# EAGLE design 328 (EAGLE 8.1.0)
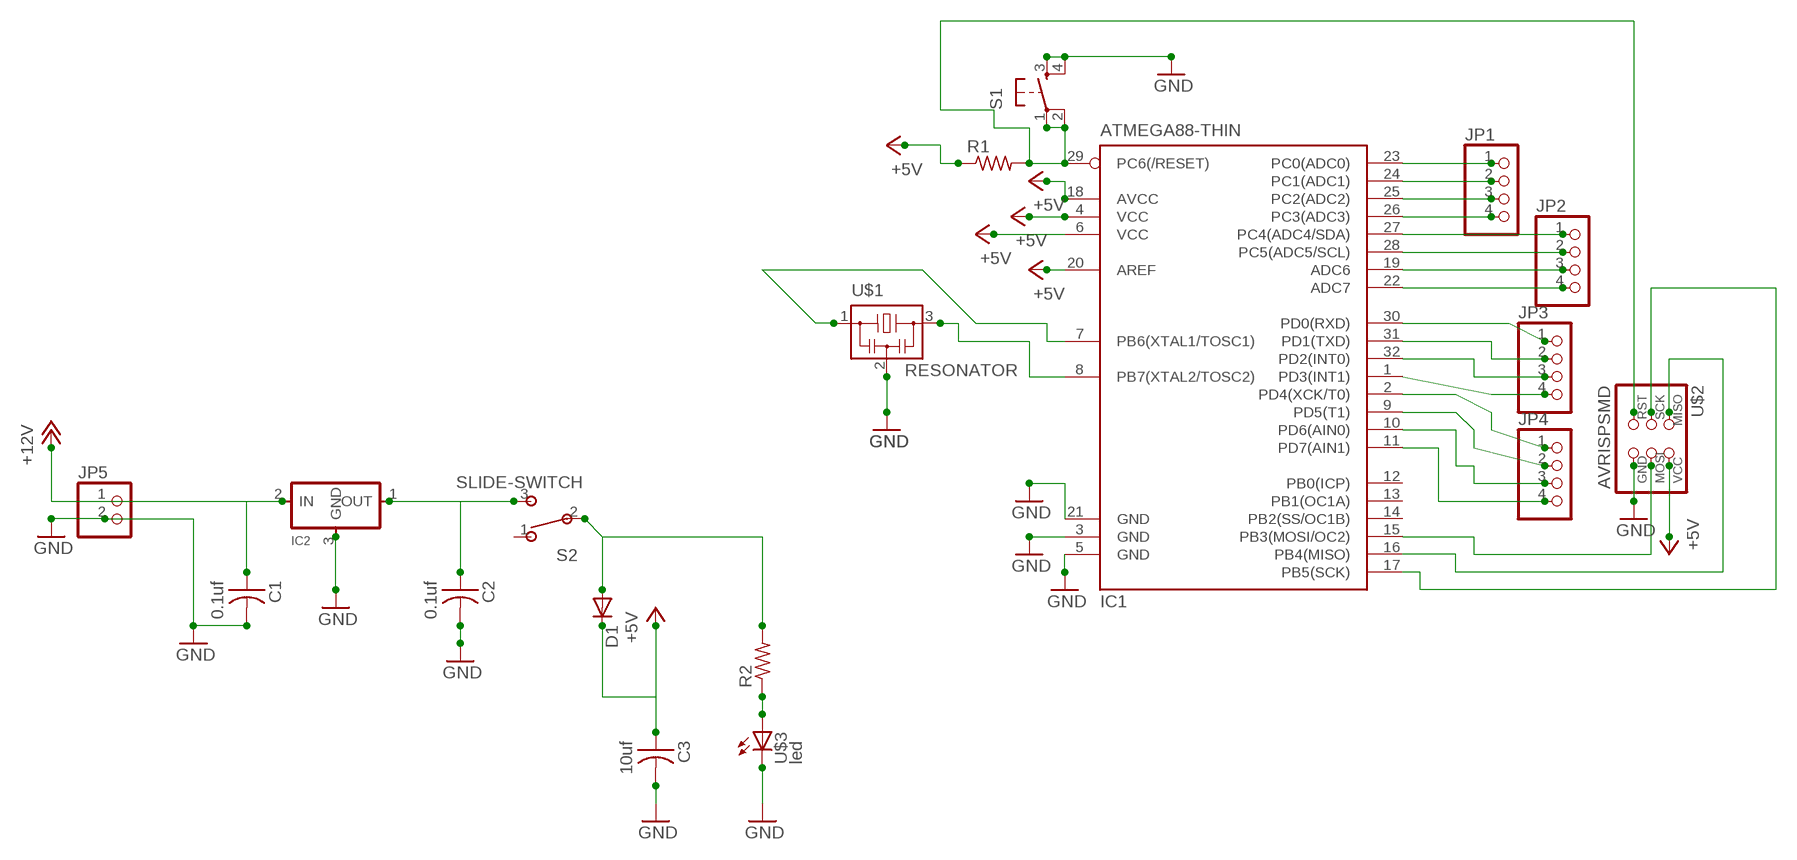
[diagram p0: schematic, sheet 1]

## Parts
C1  0.1uf  CAP-US1206FAB  [C1206FAB]
C2  0.1uf  CAP-US1206FAB  [C1206FAB]
C3  10uf  CAP-US1206FAB  [C1206FAB]
D1  DIODESOD123  [SOD123]
IC1  ATMEGA88-THIN  [TQFP32-08THIN]
IC2  REGULATORSOT23  [SOT23]
JP1  PINHD-1X4  [1X04]
JP2  PINHD-1X4  [1X04]
JP3  PINHD-1X4  [1X04]
JP4  PINHD-1X4  [1X04]
JP5  PINHD-1X2  [1X02]
R1  RES-US1206FAB  [R1206FAB]
R2  RES-US1206FAB  [R1206FAB]
S1  6MM_SWITCH6MM_SWITCH  [6MM_SWITCH]
S2  SLIDE-SWITCH  [AYZ0102AGRLC]
U$1  RESONATOR  [EFOBM]
U$2  AVRISPSMD  [2X03SMD]
U$3  led  LEDFAB1206  [LED1206FAB]

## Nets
+5V: C3.1 D1.CATHODE(C) IC1.4(VCC) IC1.6(VCC) IC1.18(AVCC) IC1.20(AREF) R1.1 U$2.2(VCC)
+12V: C1.1 IC2.2(IN) JP5.1
GND: C1.2 C2.2 C3.2 IC1.3(GND) IC1.5(GND) IC1.21(GND) IC2.3(GND) JP5.2 S1.3(S) S1.4(S1) U$1.2 U$2.6(GND) U$3.2(C)
N$1: IC1.7(PB6(XTAL1/TOSC1)) U$1.1
N$2: IC1.8(PB7(XTAL2/TOSC2)) U$1.3
N$3: IC1.29(PC6(/RESET)) R1.2 S1.1(P) S1.2(P1) U$2.5(RST)
N$4: IC1.17(PB5(SCK)) U$2.3(SCK)
N$5: IC1.16(PB4(MISO)) U$2.1(MISO)
N$6: IC1.15(PB3(MOSI/OC2)) U$2.4(MOSI)
N$7: IC1.23(PC0(ADC0)) JP1.1
N$8: IC1.24(PC1(ADC1)) JP1.2
N$9: IC1.25(PC2(ADC2)) JP1.3
N$10: IC1.26(PC3(ADC3)) JP1.4
N$11: IC1.27(PC4(ADC4/SDA)) JP2.1
N$12: IC1.28(PC5(ADC5/SCL)) JP2.2
N$13: IC1.19(ADC6) JP2.3
N$14: IC1.22(ADC7) JP2.4
N$15: IC1.30(PD0(RXD)) JP3.1
N$16: IC1.31(PD1(TXD)) JP3.2
N$17: IC1.32(PD2(INT0)) JP3.3
N$18: IC1.1(PD3(INT1)) JP3.4
N$19: IC1.2(PD4(XCK/T0)) JP4.1
N$20: IC1.9(PD5(T1)) JP4.2
N$21: IC1.10(PD6(AIN0)) JP4.3
N$22: IC1.11(PD7(AIN1)) JP4.4
N$23: D1.ANODE(A) R2.2 S2.2
N$25: R2.1 U$3.1(A)
N$27: C2.1 IC2.1(OUT) S2.3
Unconnected: IC1.12(PB0(ICP)) IC1.13(PB1(OC1A)) IC1.14(PB2(SS/OC1B)) S2.1

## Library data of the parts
C1-C3 = fab:CAP-US
D1 = fab:DIODE: DIODE
IC1 = fab:ATMEGA88-THIN
IC2 = fab:REGULATOR
JP1-JP4 = pinhead:PINHD-1X4: PIN HEADER
JP5 = pinhead:PINHD-1X2: PIN HEADER
R1 R2 = fab:RES-US: Resistor (US Symbol)
S1 = fab:6MM_SWITCH: OMRON SWITCH
S2 = fab:SLIDE-SWITCH: SMD slide-switch AYZ0102AGRLC as found in the fablab inventory. Includes the mounting holes. Made by Zaerc.
U$1 = fab:RESONATOR
U$2 = fab:AVRISP
U$3 = fab:LED: LED

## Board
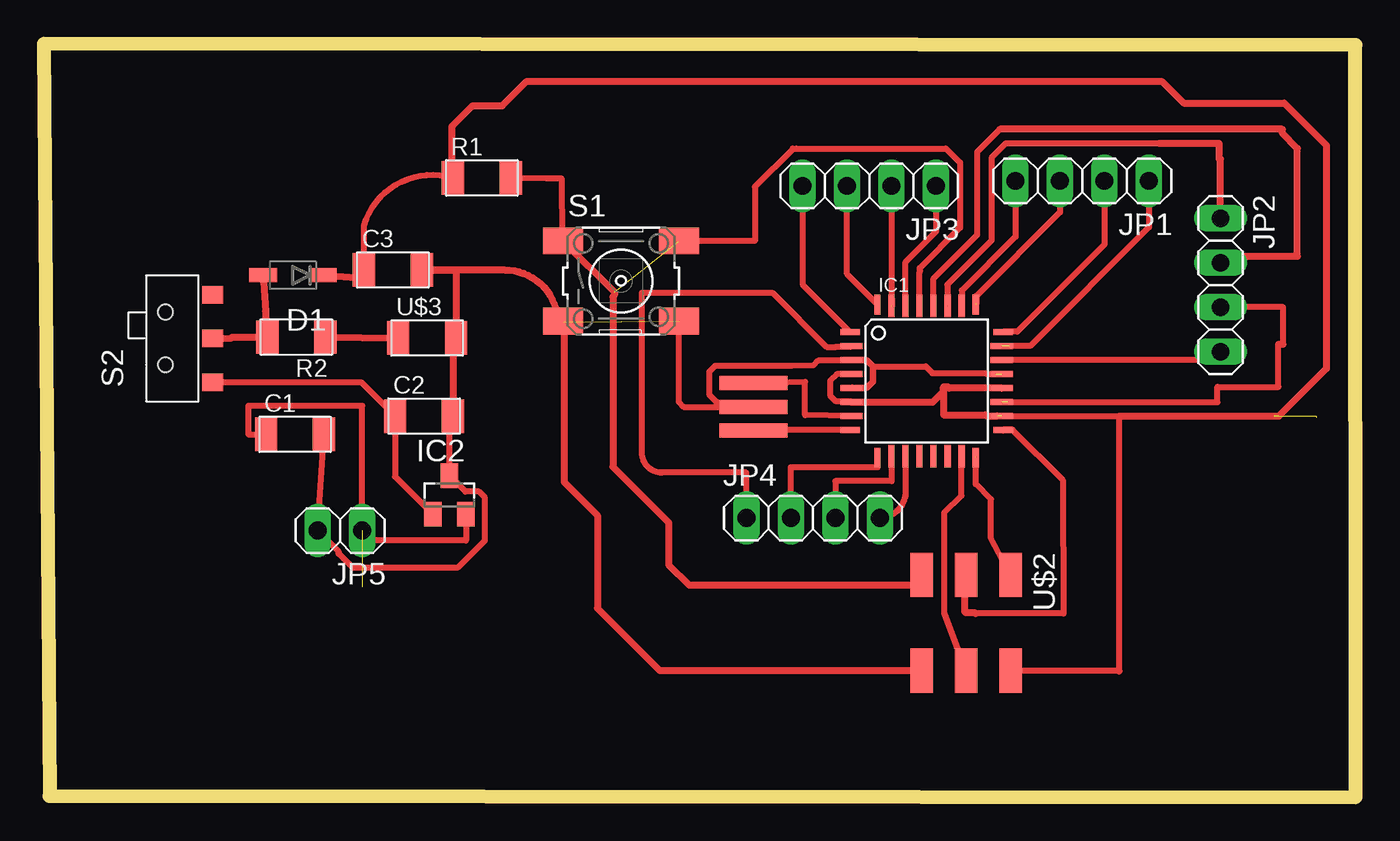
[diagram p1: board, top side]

Size 74.93 x 43.04 mm. Coordinates in mm from the lower left corner, seen from the top.
Outline: 0.33,0.08 74.93,0 74.91,42.97 0,43.04 0.33,0.08
Copper layers (1*16): Top 0.035mm / dielectric 1.5mm / Bottom 0.035mm
Design rules "default *": minimum track width 16mil, minimum drill 24mil, track to track 16mil, track to pad 16mil, pad to pad 16mil, via to via 16mil, smd to smd 8mil, copper to edge 40mil, drill to drill 8mil, minimum pad ring 10mil, minimum via ring 8mil, stop-mask expansion 4mil, vias tented up to drill 0mil, thermal gap 10mil

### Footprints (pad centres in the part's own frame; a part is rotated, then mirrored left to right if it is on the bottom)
C1206FAB = smd 1.27 x 1.905: 1 -1.651,0; 2 1.651,0
SOD123 = smd 1.6 x 0.8: ANODE 1.7,0; CATHODE -1.7,0
TQFP32-08THIN = smd 1.118 x 0.356: 1 -4.369,2.8; 8 -4.369,-2.8; 17 4.369,-2.8; 24 4.369,2.8 | smd 1.27 x 0.356: 2 -4.293,2; 3 -4.293,1.2; 4 -4.293,0.4; 5 -4.293,-0.4; 6 -4.293,-1.2; 7 -4.293,-2; 18 4.293,-2; 19 4.293,-1.2; 20 4.293,-0.4; 21 4.293,0.4; 22 4.293,1.2; 23 4.293,2 | smd 0.356 x 1.118: 9 -2.8,-4.369; 16 2.8,-4.369; 25 2.8,4.369; 32 -2.8,4.369 | smd 0.356 x 1.27: 10 -2,-4.293; 14 1.2,-4.293; 15 2,-4.293; 26 2,4.293; 27 1.2,4.293; 31 -2,4.293 | smd 0.35 x 1.27: 11 -1.2,-4.293; 12 -0.4,-4.293; 13 0.4,-4.293; 28 0.4,4.293; 29 -0.4,4.293; 30 -1.2,4.293
SOT23 = smd 1 x 1.4: 1 -0.95,-1.1; 2 0.95,-1.1; 3 0,1.1
1X04 = drill 1.016 long: 1 -3.81,0; 2 -1.27,0; 3 1.27,0; 4 3.81,0
1X02 = drill 1.016 long: 1 -1.27,0; 2 1.27,0
R1206FAB = smd 1.27 x 1.905: 1 -1.651,0; 2 1.651,0
6MM_SWITCH = smd 2.286 x 1.524: 1 -3.302,2.286; 2 3.302,2.286; 3 -3.302,-2.286; 4 3.302,-2.286
AYZ0102AGRLC = smd 1 x 1.2: 1 2.5,-2.3; 2 0,-2.3; 3 -2.5,-2.3 | hole 0.85: -1.5,0.4; 1.5,0.4
EFOBM = smd 0.8 x 3.9: 1 -1.35,0; 2 0,0; 3 1.35,0
2X03SMD = smd 2.54 x 1.27: 1 -2.54,2.54; 2 2.92,2.54; 3 -2.54,0; 4 2.92,0; 5 -2.54,-2.54; 6 2.92,-2.54
LED1206FAB = smd 1.27 x 1.905: 1 -1.651,0; 2 1.651,0

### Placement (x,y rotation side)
C1  14.35,20.73 0 top
C2  21.72,21.77 0 top
C3  19.94,30.12 0 top
D1  14.22,29.82 180 top
IC1  50.42,23.77 0 top
IC2  23.16,17.27 0 top
JP1  59.31,35.2 180 top
JP2  67.21,29.26 270 top
JP3  47.14,34.92 180 top
JP4  43.94,15.95 0 top
JP5  16.92,15.24 180 top
R1  25.02,35.38 0 top
R2  14.43,26.29 180 top
S1  32.97,29.49 0 top
S2  7.34,26.21 90 top
U$1  40.54,22.3 270 top
U$2  52.68,10.16 270 top
U$3  21.89,26.24 0 top

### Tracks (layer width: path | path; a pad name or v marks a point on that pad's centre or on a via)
+5V  (4 unrouted)
  Top 0.356: IC1.6 46.09,22.61 45.25,22.61 44.91,22.95 44.91,23.79 45.29,24.17 IC1.4 | 17.86,29.69 arc90 C3.1 18.29,32.66 arc-90 R1.1 | 61.42,7.21 61.42,21.77 IC1.18 | U$2.2 61.39,7.24
  Top 0.406: D1.CATHODE 17.86,29.69 | R1.1 23.55,35.38 23.32,35.61 23.32,38.33 24.49,39.5 26.19,39.5 27.58,40.89 63.86,40.89 65.1,39.65 70.84,39.65 73.25,37.24 73.25,24.49 70.54,21.77 61.42,21.77 | IC1.20 51.71,23.37 51.64,23.44 51.38,23.44 51.38,23.19 | 51.38,23.19 51.38,21.84 53.77,21.84 53.82,21.79 54.45,21.79 | IC1.6 50.77,22.57 51.38,23.19 | 61.39,7.24 61.42,7.21
+12V  (1 unrouted)
  Top 0.356: IC2.2 24.11,14.66 18.01,14.66 18.01,15.24 JP5.1 18.19,22.35 11.68,22.35 11.68,20.73 C1.1
GND  (2 unrouted)
  Top 0.356: 38.43,22.3 U$1.2 | 38.43,22.3 36.55,22.3 36.27,22.58 S1.4 | 47.37,24.6 47.37,23.74 47.01,23.39 46.14,23.39 IC1.5 46.16,23.41 47,23.41 47.35,23.75 47.35,24.59 47,24.94 44.23,24.94 43.95,24.67 42.73,24.64 38.35,24.64 38,24.29 38,23.01 38.43,22.58 38.43,22.3 | 47.37,24.6 47.01,24.96 46.14,24.96 IC1.3 | 47.37,24.6 50.38,24.6 50.75,24.23 53.78,24.23 53.82,24.19 54.38,24.19 | S1.3 29.67,26.77 29.36,27.08 29.03,27.41 | U$2.6 arc-90 50.06,7.16 | 23.55,21.95 arc-90 C2.2 arc90 23.16,21.56 IC2.3 24.08,17.46 24.86,17.46 25.2,17.11 25.2,14.66 23.67,13.13 17.63,13.13 16.84,13.92 16.84,14.05 JP5.2 C1.2 15.65,20.73
  Top 0.406: 29.36,27.08 arc90 26.31,30.12 C3.2 23.55,30.12 U$3.2 23.37,26.24 C2.2 | S1.3 29.72,27.15 29.72,18.01 31.62,16.1 31.62,10.8 35.18,7.24 U$2.6
N$1
  Top 0.356: IC1.7 43.48,21.83 43.48,23.72 41.63,23.67 U$1.1
N$2
  Top 0.356: IC1.8 41.63,20.97 U$1.3
N$3  (1 unrouted)
  Top 0.356: 50.03,30.04 50.03,30.24 52.32,32.53 52.32,36.26 51.52,37.06 42.98,37.06 | 42.76,37.06 42.98,37.06 | 50.03,30.04 50.03,30 50.02,29.99 IC1.29 | 50.03,30.04 50.06,30.07 | 36.25,31.75 S1.2 40.62,31.78 40.62,34.87 42.78,37.03 42.95,37.03 42.98,37.06 | R1.2 28.7,35.36 29.57,35.36 29.59,31.85 S1.1 29.95,31.78
  Top 0.406: S1.1 32.59,28.85 32.59,28.68 32.51,28.6 32.51,18.87 35.69,15.7 35.69,13.28 36.86,12.12 50.55,12.12 50.14,12.52 U$2.5
N$4
  Top 0.356: 55.33,20.97 58.19,18.11 58.24,10.49 53.21,10.49
  Top 0.406: 55.33,20.97 IC1.17 | 53.21,10.49 53.16,10.54 52.65,10.54 52.6,10.59 52.6,12.62 U$2.3
N$5  (1 unrouted)
  Top 0.356: U$2.1 54.1,14.78 54.1,17.02 53.23,17.89 53.23,19.41
N$6
  Top 0.356: IC1.15 52.42,17.21 51.44,16.25 51.44,10.52 U$2.4
N$7  (1 unrouted)
  Top 0.356: JP1.1 63.12,32.56 56.34,25.78 55.14,25.78 55.12,25.76
N$8
  Top 0.356: JP1.2 60.58,31.57 55.6,26.59 54.81,26.59 IC1.24
N$9  (1 unrouted)
  Top 0.356: JP1.3 58.04,33.41 53.26,28.63 53.26,28.18 53.24,28.17
N$10
  Top 0.356: IC1.26 52.43,28.08 52.43,28.95 55.5,32.02 JP1.4
N$11  (1 unrouted)
  Top 0.356: 51.61,28.07 51.61,29.28 54.13,31.8 54.13,36.53 54.93,37.34 63.69,37.34 | JP2.1 67.21,33.82
  Top 0.406: 67.21,33.71 JP2.1 67.21,36.47 67.13,36.47 67.13,37.34 63.69,37.34
N$12
  Top 0.356: 54.59,38.15 53.32,36.87 53.32,32.14 50.82,29.64 IC1.28
  Top 0.406: JP2.2 67.21,30.91 71.6,30.91 71.6,37.06 70.74,37.92 70.74,38.15 54.59,38.15
N$13  (1 unrouted)
  Top 0.356: 55.06,22.57 67.03,22.57 67.03,23.44 70.51,23.44 70.51,25.88 | 70.79,25.88 70.79,27.99 JP2.3
  Top 0.406: 70.51,25.88 70.79,25.88
N$14
  Top 0.356: JP2.4 arc-90 66.73,24.97 IC1.22
N$15
  Top 0.356: IC1.30 49.22,30.58 50.98,32.33 50.98,34.9 JP3.1
N$16  (1 unrouted)
  Top 0.356: JP3.2 48.41,28.5 48.43,28.48 48.43,28.07
N$17
  Top 0.356: JP3.3 45.87,29.89 IC1.32
N$18
  Top 0.356: JP3.4 43.33,29.29 IC1.1
N$19
  Top 0.356: JP4.1 40.13,18.54 35.31,18.54 arc-90 34.16,19.69 34.16,28.83 41.61,28.83 44.7,25.73 45.24,25.73 45.25,25.74 46.09,25.74 IC1.2
N$20
  Top 0.356: IC1.9 47.62,18.85 42.65,18.85 42.65,16.05 JP4.2
N$21
  Top 0.356: IC1.10 48.42,18.06 45.21,18.06 JP4.3
N$22
  Top 0.356: IC1.11 49.22,17.52 arc-90 JP4.4
N$23
  Top 0.406: S2.2 10.74,26.24 arc-90 10.78,26.28 12.24,26.28 R2.2 arc-90 12.67,26.39 12.67,27.76 12.55,29.42 12.55,29.79 arc90 D1.ANODE
N$25
  Top 0.406: R2.1 U$3.1
N$27
  Top 0.356: IC2.1 20.07,18.32 C2.1 18.12,23.71 S2.3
